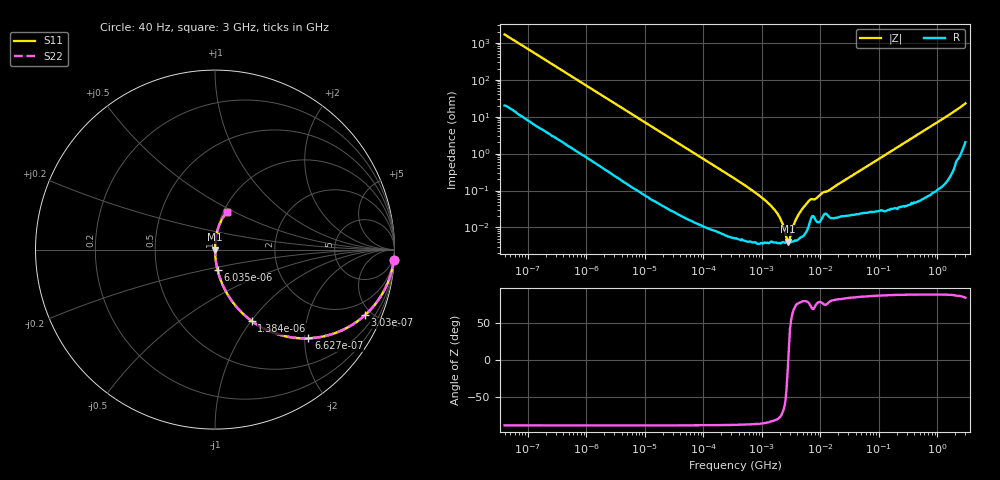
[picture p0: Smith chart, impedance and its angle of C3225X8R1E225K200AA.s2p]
! S-parameter Generated by TDK Corporation
! Copyright(C) 2015 TDK Corporation.
! All Rights Reserved.
! TDK P/N: C3225X8R1E225K200AA (Multilayer Ceramic Chip Capacitors)
! Property: C=2.2uF
! Size(LxWxT): 3.2x2.5x2mm, 0.126x0.098x0.079inches
! Model Type: s2p (Touchstone File Format Version 1.0)
! Frequency: DC=Yes Start=0.00004MHz Stop=3000MHz 396points Log-sweep
! Note: This model was converted from impedance.
! Model Generated on Jun. 23, 2015
! Hash(MD5):
! Port Assignments:
!  1 ---| |--- 2
! Applicable Conditions:
!  Temperature = 25 degC
!  DC Bias Voltage = 0 V
!  Small Signal Operation
! Terms and conditions regarding TDK Simulation Models
! (1)This simulation model is being provided solely for informational purposes. Please refer to the specifications of the products in terms of detailed characteristics of such products.
! (2)In no event shall TDK Corporation of any of its subsidiaries be liable for any loss or damage arising, directly or indirectly,
!  From any information contained in this simulation model, including, but not limited to loss or damages arising from any inaccuracies, omissions or errors in connection with such information.
! (3)Any and all copyrights on this simulation model are owned by TDK Corporation.
!  Duplication or redistribution of this simulation model without prior written permission from TDK Corporation is prohibited.
! (4)This simulation model is subject to any modification or change without any prior notice.
! (5)Neither TDK Corporation nor any of its subsidiaries shall make any warranty, express or implied,
!  Including but not limited to the correctness, implied warranties of merchantability and fitness for a particular purpose with respect to this simulation models.
! (6)The use of this simulation model shall be deemed to have consented to the terms and conditions hereof.
# MHz S MA R 50
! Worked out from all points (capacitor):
!   395 points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, 40 Hz to 3 GHz, reference 50 ohm
!   read as one part in series: C = 2.37 uF near 41.88 Hz
!   lowest |Z| = 4.15 mohm at 2.748 MHz (marker M1)
!   series resonance near 2.816 MHz, so ESL is about 1.3 nH
!   S11 on the Smith chart (normalised r, x): 40 Hz: 1, -34; 303 Hz: 1.05, -4.53; 662.7 Hz: 1.02, -2.09; 1.384 kHz: 1.01, -1.00; 6.035 kHz: 1.00, -0.23; 3 GHz: 1.04, +0.46
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4e-05  0.9975 -3.4  0.05948 85.9  0.05948 85.9  0.9975 -3.4
0.0001385867  0.9778 -11.5  0.1986 77.9  0.1986 77.9  0.9778 -11.5
0.0003030459  0.911 -23.7  0.4019 65.6  0.4019 65.6  0.911 -23.7
0.000662667  0.7177 -43.5  0.6883 45.9  0.6883 45.9  0.7177 -43.5
0.000834128  0.6351 -49.9  0.7653 39.4  0.7653 39.4  0.6351 -49.9
0.001383868  0.447 -62.8  0.8896 26.5  0.8896 26.5  0.447 -62.8
0.002635842  0.2558 -74.6  0.964 14.8  0.964 14.8  0.2558 -74.6
0.006035228  0.1159 -82.7  0.9921 6.7  0.9921 6.7  0.1159 -82.7
0.01739424  0.04084 -87.0  0.9987 2.3  0.9987 2.3  0.04084 -87.0
0.3464102  0.00207 -88.5  0.9999 0.1  0.9999 0.1  0.00207 -88.5
1.146211  0.0005372 -85.8  1 0.0  1 0.0  0.0005372 -85.8
1.816098  0.0002442 -81.1  1 0.0  1 0.0  0.0002442 -81.1
2.393669  9.489e-05 -65.6  1 0.0  1 0.0  9.489e-05 -65.6
2.748062  4.148e-05 -16.3  1 0.0  1 0.0  4.148e-05 -16.3
3.303516  9.016e-05 62.5  1 -0.0  1 -0.0  9.016e-05 62.5
4.773931  0.0003031 79.5  0.9999 -0.0  0.9999 -0.0  0.0003031 79.5
7.22376  0.0005875 69.9  0.9998 -0.0  0.9998 -0.0  0.0005875 69.9
8.293268  0.0005955 74.7  0.9998 -0.0  0.9998 -0.0  0.0005955 74.7
10.93076  0.0008697 77.2  0.9998 -0.0  0.9998 -0.0  0.0008697 77.2
150.6385  0.01083 87.8  0.9996 -0.6  0.9996 -0.6  0.01083 87.8
949.3681  0.06694 85.3  0.9968 -3.8  0.9968 -3.8  0.06694 85.3
3000  0.2188 72.3  0.9565 -12.6  0.9565 -12.6  0.2188 72.3
